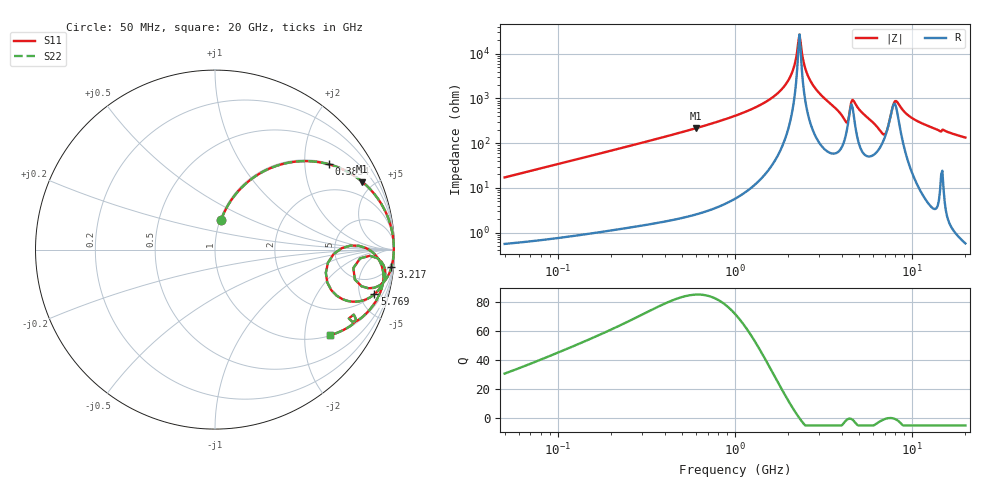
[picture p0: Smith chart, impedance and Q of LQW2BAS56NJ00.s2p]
!Murata Part Number: LQW2BAS56NJ00
!These Parameters are Measured in Series Mode Connection
!  o--[Z]--o
!Port1  Port2
!  o-------o
!Freq. Start=50[MHz] Stop=20[GHz], 401[Steps]
# Hz S RI R 50
!Freq.(Hz) S11(Real) S11(Imag) S21(Real) S21(Imag) S12(Real) S12(Imag) S22(Real) S22(Imag)
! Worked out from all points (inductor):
!   401 points, 50 MHz to 20 GHz, reference 50 ohm
!   read as one part in series: L = 54.3 nH near 51.52 MHz
!   highest Q = 85.2 at 600.9 MHz (marker M1), where L = 57.2 nH
!   self-resonance near 2.279 GHz
!   S11 on the Smith chart (normalised r, x): 50 MHz: 1.01, +0.34; 383.4 MHz: 1.03, +2.65; 3.217 GHz: 2, -20; 5.769 GHz: 2.01, -6.68; 20 GHz: 1.01, -2.67
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5e7  0.0335 0.1645  0.9665 -0.1645  0.9665 -0.1645  0.0335 0.1645
1.364002e8  0.1819 0.3763  0.8181 -0.3763  0.8181 -0.3763  0.1819 0.3763
3.721004e8  0.6213 0.4786  0.3787 -0.4786  0.3787 -0.4786  0.6213 0.4786
3.834161e8  0.6357 0.4749  0.3643 -0.4749  0.3643 -0.4749  0.6357 0.4749
6.009314e8  0.8205 0.3779  0.1795 -0.3779  0.1795 -0.3779  0.8205 0.3779
1e9  0.9408 0.2291  0.0592 -0.2291  0.0592 -0.2291  0.9408 0.2291
1.454215e9  0.9814 0.1237  0.0186 -0.1237  0.0186 -0.1237  0.9814 0.1237
1.848039e9  0.9933 0.0597  0.00669 -0.0597  0.00669 -0.0597  0.9933 0.0597
2.083303e9  0.9959 0.028  0.00412 -0.028  0.00412 -0.028  0.9959 0.028
2.313601e9  0.9963 -0.000147  0.00368 0.000147  0.00368 0.000147  0.9963 -0.000147
2.531158e9  0.9952 -0.0249  0.00476 0.0249  0.00476 0.0249  0.9952 -0.0249
2.728004e9  0.9931 -0.0464  0.00687 0.0464  0.00687 0.0464  0.9931 -0.0464
3.216634e9  0.9828 -0.0985  0.0172 0.0985  0.0172 0.0985  0.9828 -0.0985
4.212059e9  0.8166 -0.2043  0.1834 0.2043  0.1834 0.2043  0.8166 -0.2043
4.677679e9  0.9394 -0.0874  0.0606 0.0874  0.0606 0.0874  0.9394 -0.0874
5.769027e9  0.8879 -0.2489  0.1121 0.2489  0.1121 0.2489  0.8879 -0.2489
6.802353e9  0.648 -0.2259  0.352 0.2259  0.352 0.2259  0.648 -0.2259
7.442007e9  0.7554 0.0223  0.2446 -0.0223  0.2446 -0.0223  0.7554 0.0223
7.901521e9  0.8916 -0.0277  0.1084 0.0277  0.1084 0.0277  0.8916 -0.0277
8.141811e9  0.9197 -0.0684  0.0803 0.0684  0.0803 0.0684  0.9197 -0.0684
1.082228e10  0.8949 -0.2897  0.1051 0.2897  0.1051 0.2897  0.8949 -0.2897
2e10  0.6394 -0.478  0.3606 0.478  0.3606 0.478  0.6394 -0.478
